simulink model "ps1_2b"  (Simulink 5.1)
settings: Solver=ode45  StartTime=0.0  StopTime=10.0  RelTol=1e-3
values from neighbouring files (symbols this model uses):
  d22 = d(2,2)    [ps1_2.m]
libraries: cstblocks x2

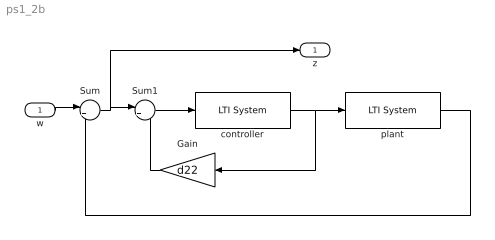
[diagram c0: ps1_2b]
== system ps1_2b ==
  w : Inport
  Gain : Gain  Orientation=left  Gain=d22
  Sum : Sum  Inputs=|+-
  Sum1 : Sum  Inputs=|+-
  controller : cstblocks/LTI System  sys=K  IC=0
  plant : cstblocks/LTI System  sys=P0  IC=[]
  z : Outport
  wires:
  w/1 -> Sum/1
  Sum/1 -> Sum1/1, z/1
  plant/1 -> Sum/2
  controller/1 -> plant/1, Gain/1
  Gain/1 -> Sum1/2
  Sum1/1 -> controller/1
